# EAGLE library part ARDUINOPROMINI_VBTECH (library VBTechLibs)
Arduino Pro Mini 3.3V
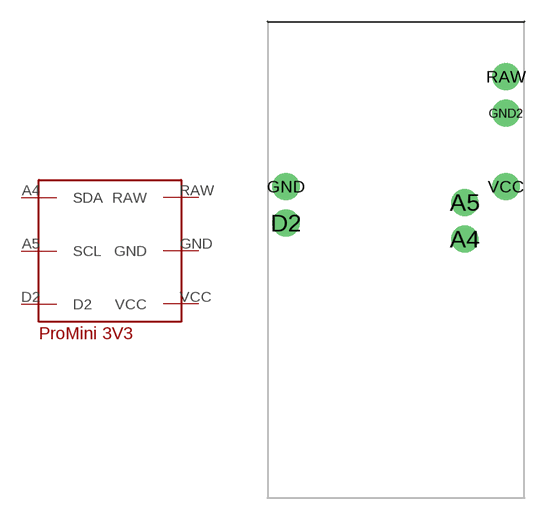
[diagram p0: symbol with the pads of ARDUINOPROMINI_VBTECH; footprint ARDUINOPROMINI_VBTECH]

Designator prefix -

## ARDUINOPROMINI_VBTECH  [ARDUINOPROMINI_VBTECH]
A4  SDA
A5  SCL
D2  D2
GND  GND
RAW  RAW
VCC  VCC

## Footprint ARDUINOPROMINI_VBTECH (pad centres in mm)
drill 1.016 pad 1.88: A4 4.763,1.429; A5 4.763,3.969; D2 -7.62,2.54; GND -7.62,5.08; GND2 7.62,10.16; RAW 7.62,12.7; VCC 7.62,5.08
